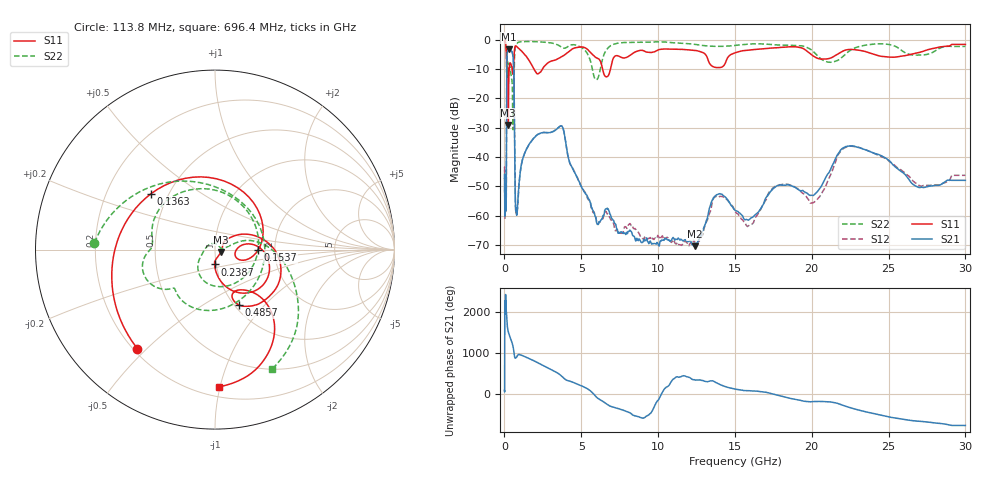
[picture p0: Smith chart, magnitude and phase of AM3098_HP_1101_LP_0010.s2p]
! Date/Time: Thu, Feb 28, 2019 8:45 AM
! Network Analyzer: Agilent Technologies E8364B Rev: A.07.50.67
! Sweep from 0.010 to 30.000 GHz, 1601 Points, Sweep Type: LOG
! Power Supply: 5.022 V, 0.002 A
# Hz S DB R 50
!freq MagS11 AngS11 MagS21 AngS21 MagS12 AngS12 MagS22 AngS22
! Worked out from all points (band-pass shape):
!   1601 points, 10 MHz to 30 GHz, reference 50 ohm
!   highest |S21| = -3.37 dB at 266.5 MHz (marker M1); lowest = -70.4 dB at 12.37 GHz (marker M2)
!   |S21| within 3 dB of the highest: 158.7 MHz to 567.3 MHz (408.6 MHz wide, 113 % of centre)
!   lowest |S11| = -29.1 dB at 250.9 MHz (marker M3), VSWR 1.07, Z = 53.3 - j1.44 ohm
!   |S11| at or under -10 dB: 206.6 MHz to 306.2 MHz (99.54 MHz wide, 38.8 % of centre); 1.909 GHz to 2.477 GHz (567.5 MHz wide, 25.9 % of centre); 6.38 GHz to 6.904 GHz (523.7 MHz wide, 7.89 % of centre)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
!   |S22| runs from -30.7 to -0.5 dB; largest |S21 - S12| = 0.01
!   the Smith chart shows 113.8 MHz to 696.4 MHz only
!   S11 on the Smith chart (normalised r, x): 113.8 MHz: 0.22, -0.47; 136.3 MHz: 0.40, +0.32; 153.7 MHz: 1.63, -0.01; 238.7 MHz: 0.98, -0.16; 485.7 MHz: 1.05, -0.72; 696.4 MHz: 0.27, -0.99
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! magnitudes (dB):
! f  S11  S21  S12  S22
! 10 MHz  -0.4  -47.3  -45.0  -0.5
! 38.04 MHz  -0.3  -57.3  -56.9  -0.6
! 113.8 MHz  -3.1  -54.4  -54.9  -3.4
! 136.3 MHz  -6.5  -25.9  -25.8  -10.6
! 144.7 MHz  -8.7  -14.2  -14.2  -10.3
! 153.7 MHz  -12.4  -7.9  -7.9  -9.3
! 238.7 MHz  -21.7  -3.5  -3.4  -8.9
! 250.9 MHz  -29.1  -3.4  -3.4  -9.1
! 266.5 MHz  -19.0  -3.4  -3.3  -9.1
! 485.7 MHz  -9.5  -4.1  -4.1  -13.8
! 550.5 MHz  -11.8  -5.6  -5.5  -29.0
! 617.6 MHz  -6.3  -13.5  -13.4  -13.7
! 696.4 MHz  -2.3  -52.1  -52.4  -2.6
! 813.3 MHz  -2.5  -59.6  -58.3  -1.2
! 2.084 GHz  -11.4  -32.7  -32.6  -0.7
! 3.723 GHz  -5.8  -29.4  -29.5  -2.6
! 5.989 GHz  -6.2  -62.2  -61.7  -13.7
! 7.926 GHz  -6.1  -66.2  -63.9  -1.0
! 12.37 GHz  -3.7  -70.4  -68.7  -1.6
! 20.2 GHz  -5.9  -52.6  -55.2  -4.6
! 22.56 GHz  -3.4  -36.2  -36.3  -3.5
! 30 GHz  -1.7  -47.9  -46.2  -2.3
